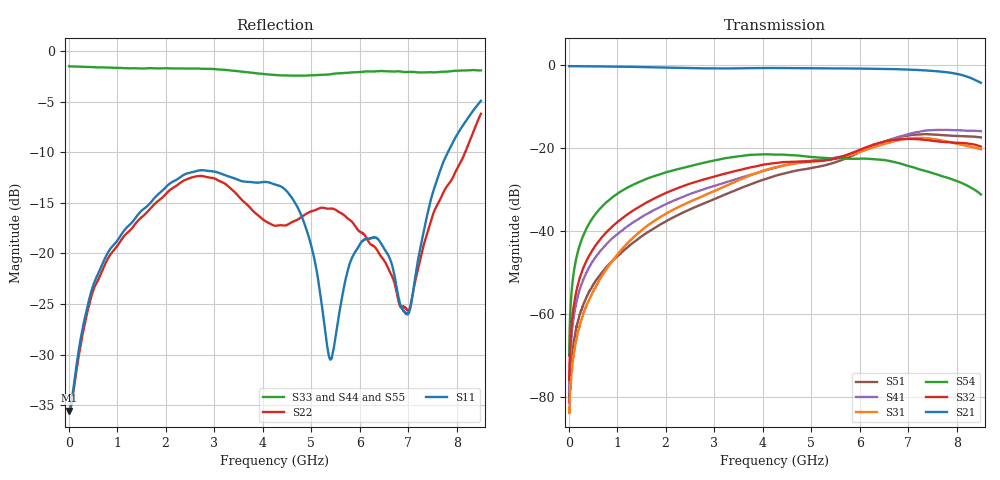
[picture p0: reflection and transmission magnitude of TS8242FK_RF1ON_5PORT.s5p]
! Created with skrf (http://scikit-rf.org).
# Hz S RI R 50.0
!freq ReS11 ImS11 ReS12 ImS12 ReS13 ImS13
! ReS14 ImS14 ReS15 ImS15
! ReS21 ImS21 ReS22 ImS22 ReS23 ImS23
! ReS24 ImS24 ReS25 ImS25
! ReS31 ImS31 ReS32 ImS32 ReS33 ImS33
! ReS34 ImS34 ReS35 ImS35
! ReS41 ImS41 ReS42 ImS42 ReS43 ImS43
! ReS44 ImS44 ReS45 ImS45
! ReS51 ImS51 ReS52 ImS52 ReS53 ImS53
! ReS54 ImS54 ReS55 ImS55
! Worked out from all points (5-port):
!   1601 points, 10 MHz to 8.5 GHz, reference 50 ohm
!   strongest paths, dB at 10 MHz, 2.132 GHz, 4.255 GHz, 6.378 GHz, 8.5 GHz:
!     S21: -0.2, -0.6, -0.6, -0.8, -4.2
!     S32: -75.7, -30.1, -23.6, -18.8, -19.6
!     S54: -69.9, -25.4, -21.5, -22.7, -31.1
!     S31: -82.8, -34.9, -24.6, -19.4, -20.2
!     S41: -78.8, -32.8, -24.7, -19.1, -15.9
!     S51: -81.2, -36.8, -26.6, -19.0, -17.4
!   lowest |S11| = -35.5 dB at 15.31 MHz (marker M1), VSWR 1.03, Z = 51.7 - j0.203 ohm
!   |S11| at or under -10 dB: start of sweep to 7.82 GHz
